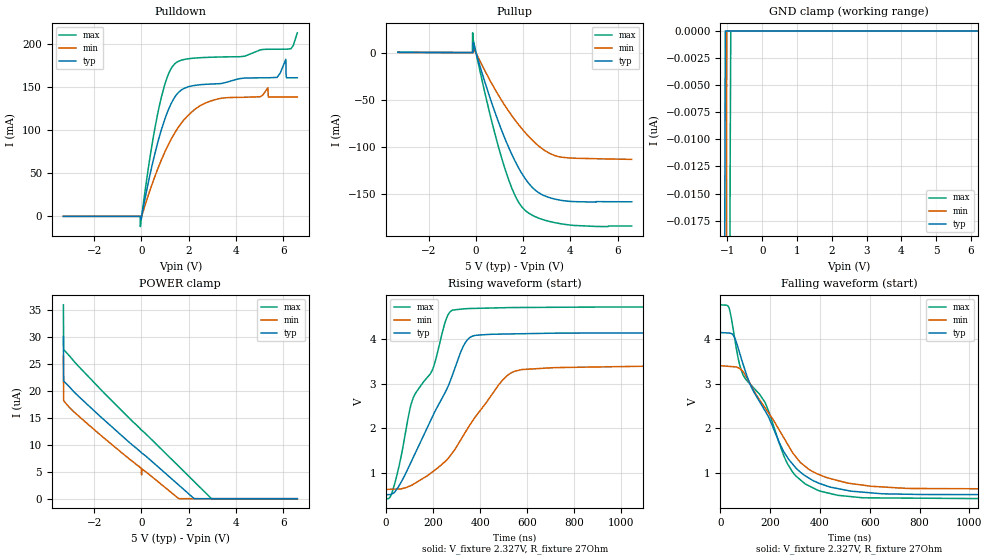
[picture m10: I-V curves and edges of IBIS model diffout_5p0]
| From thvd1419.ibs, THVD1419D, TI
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|   diffout_5p0 Model
[Model]   diffout_5p0
Model_type   I/O
Polarity   Non-Inverting
Enable   Active-High
Vinl = 0.8
Vinh = 2
Vmeas = 2.3274
Vref = 2.3274
Cref = 50pF
Rref = 27
|   typ   min   max
C_comp   801.023pF   801.023pF   801.023pF
| Where Nom  PVT is Nominal Process, 5.0V, 25C
|   Fast PVT is Strong Process,  5.5V, -40C
|   Slow PVT is Weak Process,   4.5V, 150C
[Voltage Range]   5   4.5   5.5
|Junction Temperature
[Temperature Range]   25   150   -40
[Pullup Reference]   5   4.5   5.5
[Pulldown Reference]   0   0   0
[Power Clamp Reference]   5   4.5   5.5
[GND Clamp Reference]   0   0   0
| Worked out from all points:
|   slope of the pulldown table from 0 to 0.75 V, typ, clamps not added: 8.06 ohm
|   slope of the pullup table from 0 to 0.75 V, typ, clamps not added: 12.6 ohm
|   falling waveform, V_fixture 2.327V, R_fixture 27Ohm: 20-80 % time 192ns typ, 198ns min, 201ns max; typ from 4.14 V to 0.516 V
|   rising waveform, V_fixture 2.327V, R_fixture 27Ohm: 20-80 % time 192ns typ, 226ns min, 167ns max; typ from 0.516 V to 4.14 V
[Pulldown]
|   Voltage   I(typ)   I(min)   I(max)
-3.3V     -7.501uA   -6.788uA   -8.192uA
-52.8mV   -2.982uA   -4.182uA   -2.881uA
-42.9mV   -2.964uA   -4.172uA   -11.88mA
689.7mV   85.35mA    54.8mA     118.9mA
1.343V    135.1mA    93.54mA    174.8mA
3.066V    153.7mA    135mA      184.7mA
5.353V    160.8mA    149.2mA    193.9mA
5.739V    161.2mA    138.5mA    193.9mA
6.115V    182.2mA    138.5mA    194mA
6.125V    164.6mA    138.5mA    194mA
6.145V    160.8mA    138.5mA    194mA
6.6V      160.8mA    138.5mA    213mA
[GND Clamp]
|   Voltage   I(typ)   I(min)   I(max)
-3.3V     -21.95uA   -24.24uA   -23.73uA
-1.082V   -26.83nA   -315.3nA   -1uA
-1.063V   0A         -185.5nA   -875.5nA
-1.033V   0A         -27.79nA   -689nA
-1.023V   0A         0A         -627nA
-924mV    0A         0A         -14.01nA
-904.2mV  0A         0A         0A
6.6V      0A         0A         0A
[Pullup]
|   Voltage   I(typ)   I(min)   I(max)
-3.3V     326.7uA    208.5uA    521.6uA
-141.9mV  86.09uA    72.24uA    97.76uA
-132mV    85.18uA    71.34uA    21.13mA
-112.2mV  83.34uA    69.53uA    14.55mA
-102.3mV  10.55mA    68.61uA    13.36mA
-82.5mV   7.895mA    5.187mA    10.98mA
986.7mV   -75.51mA   -46.41mA   -102.7mA
1.541V    -109.1mA   -67.61mA   -145.2mA
1.957V    -128.9mA   -81.09mA   -164.4mA
2.64V     -148.7mA   -98.91mA   -176mA
3.482V    -156.6mA   -110.6mA   -181.7mA
6.6V      -158.8mA   -113.6mA   -184.6mA
[POWER Clamp]
|   Voltage   I(typ)   I(min)   I(max)
-3.3V     30.03uA    26.43uA    35.86uA
-3.29V    21.78uA    18.16uA    27.62uA
-3.26V    21.65uA    17.99uA    27.47uA
-1.855V   15.68uA    12.24uA    20.83uA
-82.5mV   8.853uA    5.958uA    13.11uA
-3.3mV    8.525uA    5.617uA    12.72uA
6.6mV     8.487uA    4.398uA    12.69uA
16.5mV    8.455uA    5.519uA    12.65uA
1.581V    2.529uA    6.524nA    6.004uA
2.234V    4.365nA    0A         3.172uA
2.967V    0A         0A         1.739nA
6.6V      0A         0A         0A
[Ramp]
R_load = 27
|   typ   min   max
dV/dt_r   2.17407/1.90601e-07   1.65842/2.25438e-07   2.59818/1.66697e-07
dV/dt_f   2.17407/1.91019e-07   1.65842/1.96542e-07   2.59817/2.01264e-07
[Falling Waveform]
V_fixture = 2.327V
V_fixture_min = 2.016V
V_fixture_max = 2.591V
R_fixture = 27Ohm
C_fixture = 0F
|   Time   V(typ)   V(min)   V(max)
0s        4.14V      3.399V     4.757V
34.4ns    4.129V     3.384V     4.691V
54.99ns   4.049V     3.375V     4.079V
87.68ns   3.487V     3.288V     3.235V
178.7ns   2.394V     2.461V     2.583V
254.9ns   1.473V     1.784V     1.381V
289.5ns   1.202V     1.456V     1.024V
388.4ns   789.8mV    982.5mV    621.7mV
568.2ns   574.8mV    732.8mV    449.4mV
10us      516.5mV    634.8mV    427.2mV
[Rising Waveform]
V_fixture = 2.327V
V_fixture_min = 2.016V
V_fixture_max = 2.591V
R_fixture = 27Ohm
C_fixture = 0F
|   Time   V(typ)   V(min)   V(max)
0s        516.5mV    634.8mV    427.2mV
37.59ns   583.4mV    640.9mV    781.2mV
114.7ns   1.341V     745.9mV    2.673V
198.6ns   2.278V     1.032V     3.327V
261.8ns   2.92V      1.317V     4.522V
330.2ns   3.853V     1.855V     4.67V
375.3ns   4.073V     2.226V     4.68V
516.7ns   4.108V     3.186V     4.697V
726.3ns   4.127V     3.357V     4.705V
15us      4.14V      3.399V     4.758V
